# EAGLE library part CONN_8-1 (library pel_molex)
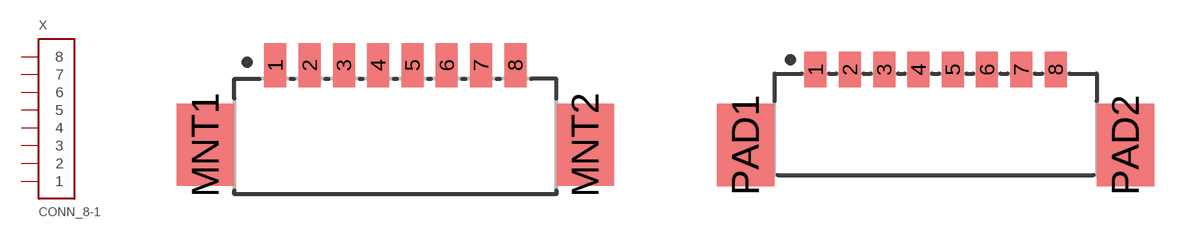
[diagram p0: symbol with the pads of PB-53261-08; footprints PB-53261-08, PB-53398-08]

Designator prefix X

## CONN_8-1-53261  [PB-53261-08]
1  1
2  2
3  3
4  4
5  5
6  6
7  7
8  8

## CONN_8-1-53398  [PB-53398-08]
Pads as for PB-53261-08

## CONN_8-1-53047  [PB-53047-08]
Pads as for PB-53261-08

## Footprint PB-53261-08 (pad centres in mm)
smd 0.8 x 1.6: 1 -4.375,1.1; 2 -3.125,1.1; 3 -1.875,1.1; 4 -0.625,1.1; 5 0.625,1.1; 6 1.875,1.1; 7 3.125,1.1; 8 4.375,1.1
smd 2.1 x 3: MNT1 -6.925,-1.8; MNT2 6.925,-1.8

## Footprint PB-53398-08 (pad centres in mm)
smd 0.8 x 1.3: 1 -4.375,1.25; 2 -3.125,1.25; 3 -1.875,1.25; 4 -0.625,1.25; 5 0.625,1.25; 6 1.875,1.25; 7 3.125,1.25; 8 4.375,1.25
smd 2.1 x 3: PAD1 -6.925,-1.5; PAD2 6.925,-1.5

## Footprint PB-53047-08 (pad centres in mm)
drill 0.5: 1 -4.375,0; 2 -3.125,0; 3 -1.875,0; 4 -0.625,0; 5 0.625,0; 6 1.875,0; 7 3.125,0; 8 4.375,0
